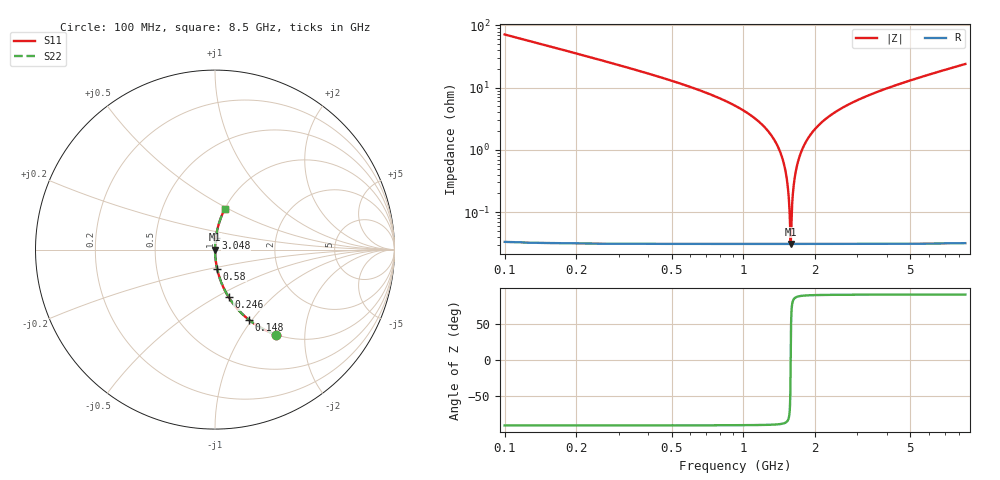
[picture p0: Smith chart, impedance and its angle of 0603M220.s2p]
! Created Wed Apr 18 16:44:44 2012
# hz S ma R 50
! 2 Port Network Data from SP1.SP block
! freq  magS11  angS11  magS21  angS21  magS12  angS12  magS22  angS22
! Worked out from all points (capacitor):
!   8401 points, 100 MHz to 8.5 GHz, reference 50 ohm
!   read as one part in series: C = 22.1 pF near 142 MHz
!   lowest |Z| = 30.8 mohm at 1.577 GHz (marker M1)
!   series resonance near 1.577 GHz, so ESL is about 460 pH
!   S11 on the Smith chart (normalised r, x): 100 MHz: 1.00, -1.43; 148 MHz: 1.00, -0.96; 246 MHz: 1.00, -0.57; 580 MHz: 1.00, -0.21; 3.048 GHz: 1.00, +0.13; 8.5 GHz: 1.00, +0.48
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1e8  0.5827 -54.3  0.8124 35.6  0.8124 35.6  0.5827 -54.3
1.48e8  0.4343 -64.2  0.9005 25.7  0.9005 25.7  0.4343 -64.2
2.46e8  0.2746 -74.0  0.9613 15.9  0.9613 15.9  0.2746 -74.0
5.8e8  0.1067 -83.7  0.994 6.1  0.994 6.1  0.1067 -83.7
1.246e9  0.02171 -87.9  0.9995 1.2  0.9995 1.2  0.02171 -87.9
1.406e9  0.01051 -87.7  0.9996 0.6  0.9996 0.6  0.01051 -87.7
1.5e9  0.004581 -85.9  0.9997 0.3  0.9997 0.3  0.004581 -85.9
1.521e9  0.003314 -84.5  0.9997 0.2  0.9997 0.2  0.003314 -84.5
1.549e9  0.001661 -79.2  0.9997 0.1  0.9997 0.1  0.001661 -79.2
1.577e9  0.0003078 0.7  0.9997 -0.0  0.9997 -0.0  0.0003078 0.7
1.602e9  0.001473 77.9  0.9997 -0.1  0.9997 -0.1  0.001473 77.9
1.643e9  0.003763 85.1  0.9997 -0.2  0.9997 -0.2  0.003763 85.1
1.693e9  0.0065 86.9  0.9997 -0.4  0.9997 -0.4  0.0065 86.9
1.773e9  0.01073 87.7  0.9996 -0.6  0.9996 -0.6  0.01073 87.7
1.886e9  0.01644 88.0  0.9996 -0.9  0.9996 -0.9  0.01644 88.0
2.269e9  0.03397 87.5  0.9991 -1.9  0.9991 -1.9  0.03397 87.5
2.9e9  0.05912 86.3  0.9979 -3.4  0.9979 -3.4  0.05912 86.3
3.048e9  0.06459 86.0  0.9976 -3.7  0.9976 -3.7  0.06459 86.0
4.3e9  0.1075 83.7  0.9939 -6.2  0.9939 -6.2  0.1075 83.7
5.7e9  0.1515 81.2  0.9882 -8.7  0.9882 -8.7  0.1515 81.2
7.1e9  0.1935 78.8  0.9808 -11.2  0.9808 -11.2  0.1935 78.8
8.5e9  0.2341 76.4  0.9719 -13.5  0.9719 -13.5  0.2341 76.4
